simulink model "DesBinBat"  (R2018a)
settings: Solver=VariableStepAuto  StartTime=0.0  StopTime=500  RelTol=1e-3
undefined symbols (not defined in the file): a7aa, b2962b33, DesBinBat, ed1d92956731, fb6c4419, sdiscope

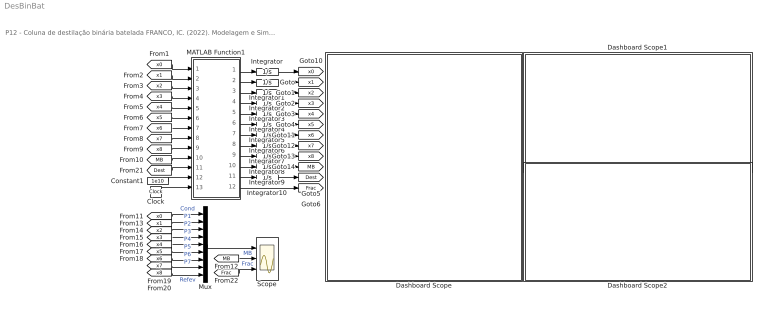
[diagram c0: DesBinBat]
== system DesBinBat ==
  note: P12 - Coluna de destilação binária batelada FRANCO, IC. (2022). Modelagem e Simulação: Problemas Típicos da Engenharia Química para Simulação e Análise. NOTAS DE AULA INOVADORAS. The Journal of Engineering and Exact Sciences. Material Complementar.
  Clock : Clock
  Constant1 : Constant  Value=1e10
  Dashboard Scope : Subsystem  DialogController=hmiCreateDDGDialog  IsWebBlock=on  mask(MWDashboardBlock){webBlockId=b2962b33-9662-4c9c-8271-65e068440fd5, webBlockType=sdiscope, ShowInitialText=on, HMISrcModelName=DesBinBat}
      mask prompts: webBlockId "WebBlock Id"; webBlockType "WebBlock Type"; HMISrcModelName "Source Model"
      mask help: SimulinkHMI:dialogs:HMIScopeDialogDesc
  Dashboard Scope1 : Subsystem  DialogController=hmiCreateDDGDialog  IsWebBlock=on  mask(MWDashboardBlock){webBlockId=fb6c4419-710d-48be-a7aa-ed1d92956731, webBlockType=sdiscope, ShowInitialText=on, HMISrcModelName=DesBinBat}
      mask prompts: webBlockId "WebBlock Id"; webBlockType "WebBlock Type"; HMISrcModelName "Source Model"
      mask help: SimulinkHMI:dialogs:HMIScopeDialogDesc
  Dashboard Scope2 : Subsystem  DialogController=hmiCreateDDGDialog  IsWebBlock=on  mask(MWDashboardBlock){webBlockId=5af55c7c-dcd2-4623-bbe8-5e8f638c5b8e, webBlockType=sdiscope, ShowInitialText=on, HMISrcModelName=DesBinBat}
      mask prompts: webBlockId "WebBlock Id"; webBlockType "WebBlock Type"; HMISrcModelName "Source Model"
      mask help: SimulinkHMI:dialogs:HMIScopeDialogDesc
  Integrator : Integrator  InitialCondition=0.9
  Integrator{1..7,10} (8 alike) : Integrator
  Integrator8 : Integrator  InitialCondition=0.8
  Integrator9 : Integrator  InitialCondition=2500
  MATLAB Function1 : MATLAB Function  TreatAsAtomicUnit=on
  Mux : Mux  Inputs=9
  Scope : Scope  NumInputPorts=3
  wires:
  MATLAB Function1/1(dx0) -> Integrator/1
  Integrator/1 -> [x0]
  [x0] -> MATLAB Function1/1(x0)
  MATLAB Function1/2(dx1) -> Integrator1/1
  Integrator1/1 -> [x1]
  [x1] -> MATLAB Function1/2(x1)
  [x2] -> MATLAB Function1/3(x2)
  MATLAB Function1/3(dx2) -> Integrator2/1
  Integrator2/1 -> [x2]
  [x3] -> MATLAB Function1/4(x3)
  MATLAB Function1/4(dx3) -> Integrator3/1
  Integrator3/1 -> [x3]
  MATLAB Function1/5(dx4) -> Integrator4/1
  Integrator4/1 -> [x4]
  [x4] -> MATLAB Function1/5(x4)
  MATLAB Function1/6(dx5) -> Integrator5/1
  Integrator5/1 -> [x5]
  [x5] -> MATLAB Function1/6(x5)
  MATLAB Function1/7(dx6) -> Integrator6/1
  Integrator6/1 -> [x6]
  [x6] -> MATLAB Function1/7(x6)
  MATLAB Function1/8(dx7) -> Integrator7/1
  [x7] -> MATLAB Function1/8(x7)
  Integrator7/1 -> [x7]
  MATLAB Function1/9(dx8) -> Integrator8/1
  Integrator8/1 -> [x8]
  [x8] -> MATLAB Function1/9(x8)
  Integrator9/1 -> [MB]
  MATLAB Function1/10(dMB) -> Integrator9/1
  Constant1/1 -> MATLAB Function1/12(R)
  [x3] -> Mux/4  "P3"
  [x5] -> Mux/6  "P5"
  [x8] -> Mux/9  "Refev"
  [x2] -> Mux/3  "P2"
  [x0] -> Mux/1  "Cond"
  [x7] -> Mux/8  "P7"
  [x6] -> Mux/7  "P6"
  [x1] -> Mux/2  "P1"
  [x4] -> Mux/5  "P4"
  Mux/1 -> Scope/1
  [MB] -> MATLAB Function1/10(MB)
  MATLAB Function1/11(dDest) -> Integrator10/1
  Integrator10/1 -> [Dest]
  [Dest] -> MATLAB Function1/11(Dest)
  MATLAB Function1/12(Frac) -> [Frac]
  [Frac] -> Scope/3  "Frac"
  Clock/1 -> MATLAB Function1/13(t)
  [MB] -> Scope/2  "MB"

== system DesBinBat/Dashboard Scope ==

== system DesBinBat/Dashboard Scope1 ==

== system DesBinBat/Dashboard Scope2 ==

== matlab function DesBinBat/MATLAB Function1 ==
function [dx0,dx1,dx2,dx3,dx4,dx5,dx6,dx7,dx8,dMB,dDest,Frac]=fcn(x0,x1,x2,x3,x4,x5,x6,x7,x8,MB,Dest,R,t)
%% Parâmetros
M     =  20.00;
M0    = 100.00;
MB0   =2500.00;
V     =  10.00;
alpha =   3.50;

%% Iniciando o processo em refluxo total
if t>75
   R=0.25;
end
if t>150
    R=1.00;
end
if t>250
    R=5.00;
end
if t>350
    R=50.00;
end

%% equações auxiliares
% vazões molares
D = V/(R+1);
L = V-D;

% equilíbrio líquido-vapor
y1=alpha*x1/(1+(alpha-1)*x1);
y2=alpha*x2/(1+(alpha-1)*x2);
y3=alpha*x3/(1+(alpha-1)*x3);
y4=alpha*x4/(1+(alpha-1)*x4);
y5=alpha*x5/(1+(alpha-1)*x5);
y6=alpha*x6/(1+(alpha-1)*x6);
y7=alpha*x7/(1+(alpha-1)*x7);
y8=alpha*x8/(1+(alpha-1)*x8);

% fração de destilado
Frac=Dest/MB0;

%% Modelo matemático
% concensador
dx0=(1/M0)*(V*y1-(L+D)*x0);
% pratos 1 a 7
dx1=(1/M)*(L*(x0-x1)+V*(y2-y1));
dx2=(1/M)*(L*(x1-x2)+V*(y3-y2));
dx3=(1/M)*(L*(x2-x3)+V*(y4-y3));
dx4=(1/M)*(L*(x3-x4)+V*(y5-y4));
dx5=(1/M)*(L*(x4-x5)+V*(y6-y5));
dx6=(1/M)*(L*(x5-x6)+V*(y7-y6));
dx7=(1/M)*(L*(x6-x7)+V*(y8-y7));
% refervedor
dMB=L-V;
dx8=(1/MB)*(L*x7-V*y8);
% total de destilado removido
dDest =D;
end
